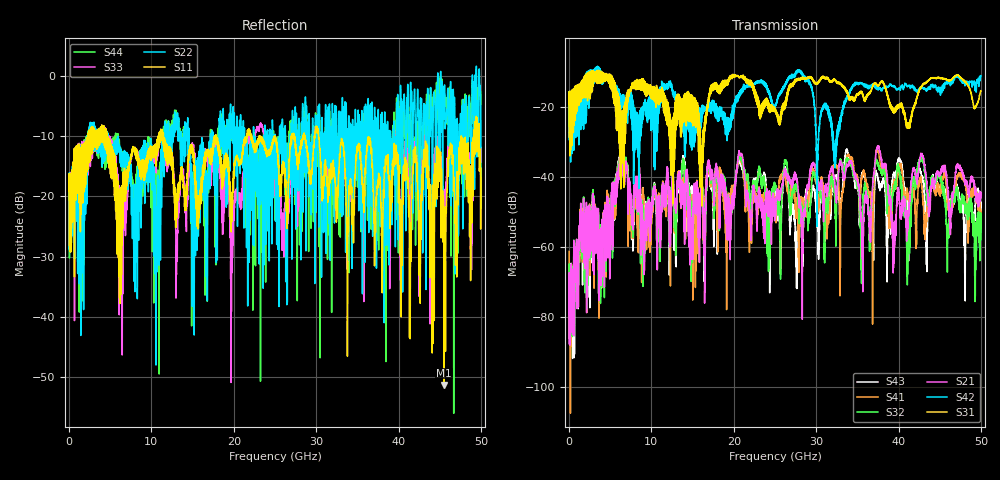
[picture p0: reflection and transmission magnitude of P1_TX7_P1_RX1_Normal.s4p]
!Keysight Technologies,N5225B,MY57041031,A.13.20.10
!Date: Friday, May 31, 2019 11:14:22
!Correction: S11(Full 4 Port(1,2,3,4))
!S12(Full 4 Port(1,2,3,4))
!S13(Full 4 Port(1,2,3,4))
!S14(Full 4 Port(1,2,3,4))
!S21(Full 4 Port(1,2,3,4))
!S22(Full 4 Port(1,2,3,4))
!S23(Full 4 Port(1,2,3,4))
!S24(Full 4 Port(1,2,3,4))
!S31(Full 4 Port(1,2,3,4))
!S32(Full 4 Port(1,2,3,4))
!S33(Full 4 Port(1,2,3,4))
!S34(Full 4 Port(1,2,3,4))
!S41(Full 4 Port(1,2,3,4))
!S42(Full 4 Port(1,2,3,4))
!S43(Full 4 Port(1,2,3,4))
!S44(Full 4 Port(1,2,3,4))
!S4P File: Measurements: <S11,S12,S13,S14>,
!<S21,S22,S23,S24>,
!<S31,S32,S33,S34>,
!<S41,S42,S43,S44>:
# Hz S  dB  R 50.0
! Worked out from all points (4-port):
!   5000 points, 10 MHz to 50 GHz, reference 50 ohm
!   strongest paths, dB at 10 MHz, 12.51 GHz, 25.01 GHz, 37.51 GHz, 50 GHz:
!     S31: -19.4, -38.8, -20.9, -14.0, -15.5
!     S42: -19.5, -14.7, -20.0, -15.1, -11.2
!     S21: -74.8, -41.0, -52.2, -31.5, -45.0
!     S32: -69.4, -41.0, -42.5, -36.2, -52.9
!     S41: -61.3, -43.3, -47.2, -32.8, -49.3
!     S43: -67.7, -42.8, -45.7, -40.5, -49.5
!   lowest |S11| = -51.3 dB at 45.52 GHz (marker M1), VSWR 1.01, Z = 49.8 + j0.195 ohm
!   |S11| at or under -10 dB: 4.613 GHz to 10.86 GHz (6.246 GHz wide, 80.7 % of centre); 11.46 GHz to 17.74 GHz (6.279 GHz wide, 43 % of centre); 30.28 GHz to 47.62 GHz (17.33 GHz wide, 44.5 % of centre)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
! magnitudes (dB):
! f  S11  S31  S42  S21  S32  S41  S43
! 10 MHz  -19.2  -19.4  -19.5  -74.8  -69.4  -61.3  -67.7
! 6.28 GHz  -24.3  -26.2  -17.8  -37.6  -36.2  -35.6  -34.5
! 8.97 GHz  -16.2  -13.8  -20.3  -59.3  -54.9  -49.1  -47.3
! 16.1 GHz  -18.0  -35.0  -22.6  -43.7  -43.6  -43.1  -43.0
! 19.84 GHz  -21.4  -11.4  -19.6  -46.2  -46.2  -43.6  -44.7
! 45.52 GHz  -51.3  -12.0  -13.8  -37.1  -43.6  -38.5  -43.6
! 50 GHz  -15.4  -15.5  -11.2  -45.0  -52.9  -49.3  -49.5
